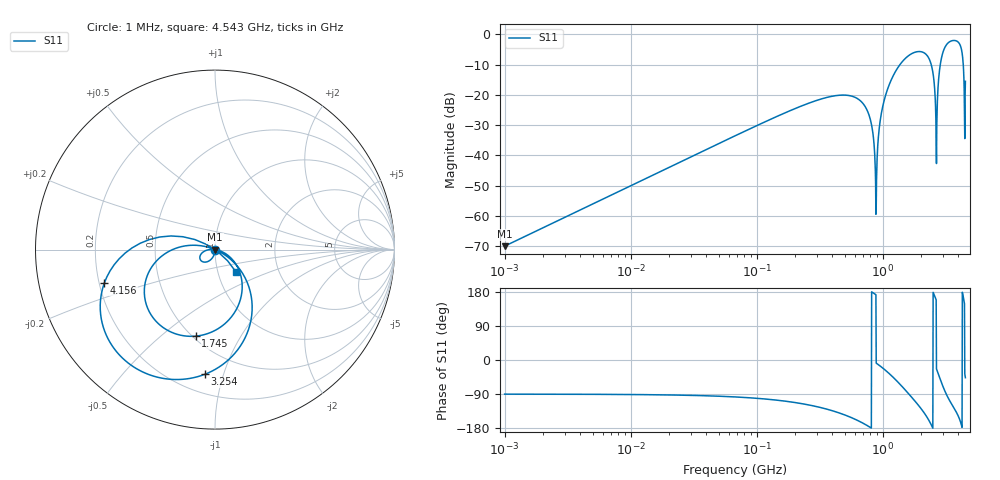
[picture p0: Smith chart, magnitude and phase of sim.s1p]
# HZ S RI R 50
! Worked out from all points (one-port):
!   1515 points, 1 MHz to 4.543 GHz, reference 50 ohm
!   lowest |S11| = -70.1 dB at 1 MHz (marker M1), VSWR 1.00, Z = 50 - j0.0314 ohm
!   |S11| at or under -10 dB: start of sweep to 1.373 GHz; 2.434 GHz to 2.871 GHz (436.9 MHz wide, 16.5 % of centre); 4.369 GHz to end of sweep
!   S11 on the Smith chart (normalised r, x): 1 MHz: 1.00, -0.00; 1.745 GHz: 0.52, -0.66; 3.254 GHz: 0.32, -0.87; 4.156 GHz: 0.22, -0.14; 4.543 GHz: 1.22, -0.31
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1000000  -6.06e-07 -0.000314
2877260  -5.01e-06 -0.000904
8232720  -4.1e-05 -0.00259
2.35563e7  -0.000336 -0.00739
6.74018e7  -0.00272 -0.0208
1.93933e8  -0.0209 -0.0534
5.549e8  -0.0844 -0.0471
7.70442e8  -0.0498 -0.00462
8.23623e8  -0.0294 0.000351
8.611e8  -0.0127 0.0011
8.85385e8  -0.00105 0.000142
9.10355e8  0.0115 -0.00213
9.62426e8  0.0387 -0.0115
1.05787e9  0.0881 -0.046
1.26397e9  0.151 -0.1896
1.58774e9  0.0243 -0.4361
1.7452e9  -0.1065 -0.482
2.34356e9  -0.3714 -0.131
2.49143e9  -0.2545 -0.00863
2.59035e9  -0.1241 0.0243
2.66341e9  -0.0152 0.00592
2.73852e9  0.0891 -0.056
2.91131e9  0.207 -0.3134
3.25388e9  -0.0573 -0.695
3.69796e9  -0.4837 -0.6319
4.15616e9  -0.6159 -0.1843
4.34528e9  -0.3648 0.0562
4.543e9  0.1153 -0.1221
